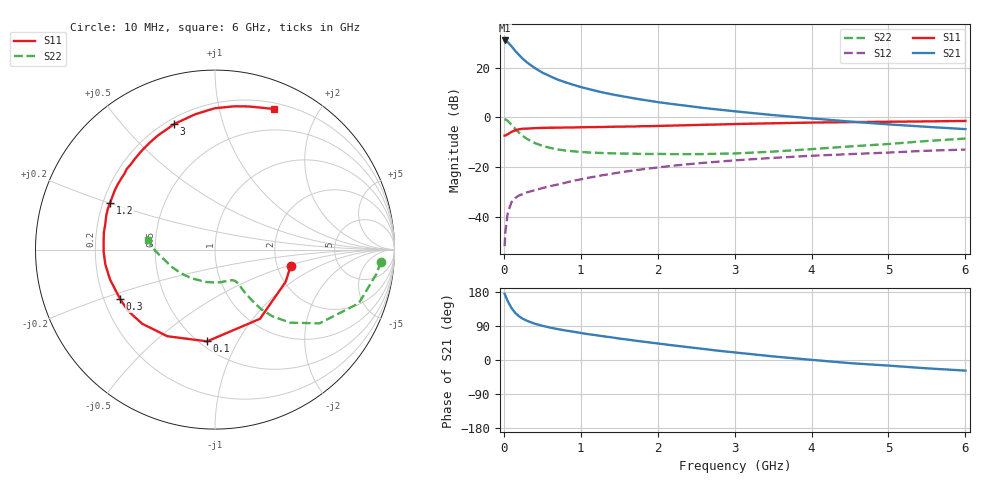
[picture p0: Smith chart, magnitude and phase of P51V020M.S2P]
! SIEMENS Small Signal Semiconductors
! BFP183
! Si NPN RF Bipolar Junction Transistor in SOT143
! VCE = 1 V  IC = 20 mA
! Common Emitter S-Parameters:  March  1996
# GHz  S  MA  R  50
!  f  S11  S21  S12  S22
! GHz  MAG  ANG  MAG  ANG  MAG  ANG  MAG  ANG
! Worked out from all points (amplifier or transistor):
!   36 points, 10 MHz to 6 GHz, reference 50 ohm
!   highest |S21| = 30.9 dB at 10 MHz (marker M1)
!   |S21| within 3 dB of that: start of sweep to 117 MHz
!   unconditionally stable (mu >= 1): 571.9 MHz to end of sweep
!   at 250 MHz: K = 0.59, MSG = 27.1 dB, |S12| = -30.7 dB
!   at 1.4 GHz: K = 1.29, MAG = 12.7 dB, |S12| = -22.6 dB
!   at 6 GHz: K = 1.06, MAG = 2.6 dB, |S12| = -12.9 dB
!   S11 on the Smith chart (normalised r, x): 10 MHz: 2.37, -0.53; 100 MHz: 0.55, -0.76; 300 MHz: 0.27, -0.23; 1.2 GHz: 0.23, +0.20; 3 GHz: 0.23, +0.70; 6 GHz: 0.26, +1.47
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0.01  0.4311 -12.2  35.07 175.0  0.0026 86.3  0.9257 -4.2
0.02  0.4328 -24.4  34.85 170.2  0.005 80.8  0.9101 -8.5
0.05  0.4599 -57.0  32.57 155.5  0.012 71.8  0.8551 -20.5
0.1  0.5131 -94.9  26.68 137.0  0.02 55.7  0.7126 -35.2
0.15  0.5508 -118.8  21.59 123.9  0.0242 49.6  0.5842 -44.2
0.2  0.5789 -134.4  17.76 115.1  0.0272 45.8  0.4898 -49.3
0.25  0.5933 -145.0  14.85 108.5  0.0291 44.6  0.4224 -52.1
0.3  0.596 -152.6  12.75 103.6  0.0313 44.0  0.3711 -53.5
0.4  0.6081 -164.1  9.844 95.9  0.0345 44.9  0.3066 -54.9
0.5  0.6165 -172.3  7.944 90.3  0.038 45.6  0.2693 -55.4
0.6  0.6203 -178.8  6.717 85.6  0.0416 47.6  0.2448 -55.5
0.7  0.6219 176.1  5.745 81.5  0.045 48.9  0.2278 -55.9
0.8  0.6266 171.2  5.071 77.9  0.0488 50.1  0.2162 -56.5
1.1  0.6385 159.4  3.721 68.1  0.0615 51.7  0.1981 -59.6
1.2  0.6403 156.0  3.401 65.4  0.0654 51.7  0.1948 -61.1
1.7  0.6578 140.2  2.404 51.3  0.0867 50.4  0.1863 -71.4
2.2  0.6858 126.5  1.847 38.6  0.1072 46.9  0.1829 -85.2
3  0.7357 108.0  1.328 20.0  0.1372 39.8  0.1888 -111.9
3.5  0.7624 98.2  1.114 9.5  0.154 35.3  0.2058 -128.9
4.5  0.8044 82.7  0.825 -8.3  0.1833 25.9  0.2614 -158.9
5.5  0.8319 71.9  0.647 -22.0  0.2143 17.5  0.3361 -179.4
6  0.8494 67.2  0.582 -28.0  0.2263 12.7  0.3761 172.1
